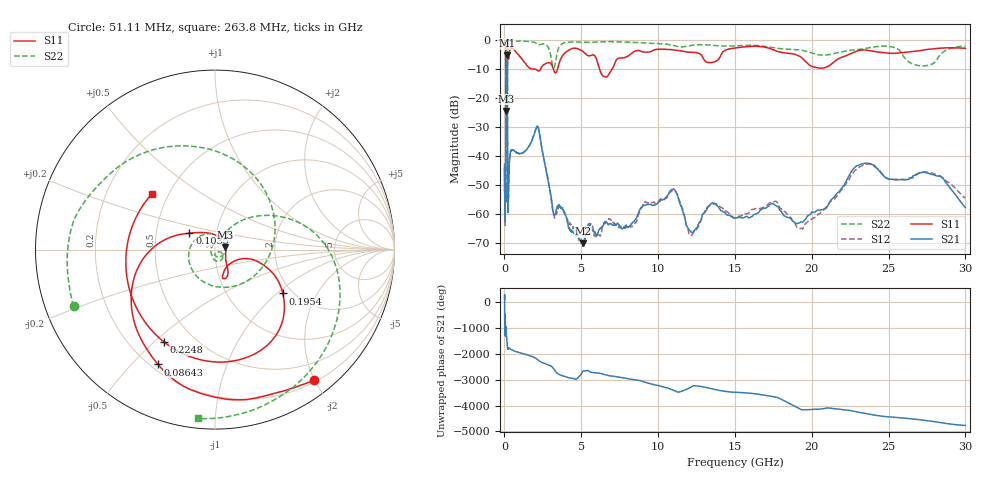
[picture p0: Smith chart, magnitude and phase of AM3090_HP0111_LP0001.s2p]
! Date/Time: Thu, Feb 28, 2019 2:00 PM
! Network Analyzer: Agilent Technologies E8364B Rev: A.07.50.67
! Sweep from 0.010 to 30.000 GHz, 1601 Points, Sweep Type: LOG
! Power Supply: 5.023 V, 0.002 A
# Hz S DB R 50
!freq MagS11 AngS11 MagS21 AngS21 MagS12 AngS12 MagS22 AngS22
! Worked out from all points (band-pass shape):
!   1601 points, 10 MHz to 30 GHz, reference 50 ohm
!   highest |S21| = -5.30 dB at 143.3 MHz (marker M1); lowest = -70.1 dB at 5.103 GHz (marker M2)
!   |S21| within 3 dB of the highest: 111.7 MHz to 179.2 MHz (67.48 MHz wide, 46.4 % of centre)
!   lowest |S11| = -24.5 dB at 109.9 MHz (marker M3), VSWR 1.13, Z = 56.2 + j1.51 ohm
!   |S11| at or under -10 dB: 1.999 GHz to 2.355 GHz (355.7 MHz wide, 16.3 % of centre); 3.186 GHz to 3.456 GHz (270.5 MHz wide, 8.15 % of centre); 6.184 GHz to 7.008 GHz (824.3 MHz wide, 12.5 % of centre)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
!   |S22| runs from -35.0 to -0.1 dB; largest |S21 - S12| = 0.012
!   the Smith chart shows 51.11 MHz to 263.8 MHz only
!   S11 on the Smith chart (normalised r, x): 51.11 MHz: 0.23, -2.00; 86.43 MHz: 0.23, -0.60; 103.5 MHz: 0.74, +0.14; 195.4 MHz: 1.79, -1.09; 224.8 MHz: 0.34, -0.54; 263.8 MHz: 0.41, +0.32
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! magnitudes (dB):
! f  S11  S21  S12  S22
! 10 MHz  -0.3  -43.3  -42.5  -0.5
! 38.04 MHz  -0.5  -59.9  -61.7  -1.3
! 51.11 MHz  -0.8  -52.8  -50.0  -1.4
! 86.43 MHz  -2.9  -49.8  -51.0  -6.2
! 103.5 MHz  -15.4  -14.9  -14.9  -15.5
! 109.9 MHz  -24.5  -9.1  -9.1  -19.4
! 143.3 MHz  -16.6  -5.3  -5.3  -32.2
! 144.7 MHz  -16.7  -5.3  -5.3  -30.1
! 172.4 MHz  -17.1  -6.9  -6.8  -32.5
! 195.4 MHz  -6.9  -22.2  -22.2  -8.3
! 224.8 MHz  -4.6  -58.8  -57.4  -1.2
! 263.8 MHz  -6.6  -52.2  -54.0  -0.5
! 550.5 MHz  -3.0  -38.0  -38.1  -0.2
! 2.084 GHz  -10.3  -30.0  -30.0  -1.2
! 3.204 GHz  -10.3  -60.1  -60.3  -9.6
! 5.103 GHz  -3.9  -70.1  -71.0  -0.8
! 7.926 GHz  -5.8  -64.2  -63.8  -0.7
! 10.86 GHz  -3.3  -51.6  -52.1  -1.7
! 12.25 GHz  -4.3  -66.5  -66.9  -1.8
! 19.51 GHz  -6.9  -62.3  -63.8  -3.7
! 23.48 GHz  -3.4  -42.5  -42.9  -2.9
! 30 GHz  -2.8  -57.8  -54.5  -2.2
